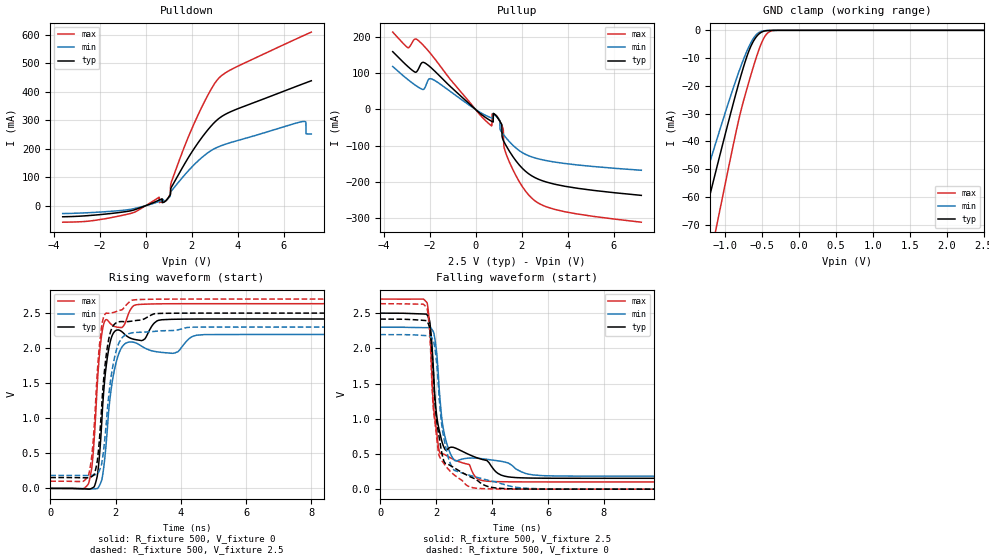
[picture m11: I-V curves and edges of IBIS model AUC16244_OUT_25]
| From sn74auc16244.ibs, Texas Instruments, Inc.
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[Model]   AUC16244_OUT_25
Model_type  3-state
Enable   Active-Low
Vref =   0
Rref =   500
Cref =   30p
Vmeas =   1.25
| variable   typ   min   max
C_comp   5.24pF   4.67pF   5.46pF
| C_pullup   7.75pF   4.60pF   11.92pF
| C_pulldown   6.72pF   4.63pF   15.60pF
| C_tri-state   5.24pF   4.67pF   5.46pF
[Temperature Range]   40   100   -40
| Ambient temperature   25   85   -40
[Voltage range]   2.5   2.3   2.7
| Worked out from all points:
|   slope of the pulldown table from 0 to 0.375 V, typ, clamps not added: 30.7 ohm
|   slope of the pullup table from 0 to 0.375 V, typ, clamps not added: 19 ohm
|   GND clamp passes 1 mA (typ) near -0.53 V on its own axis
|   rising waveform, R_fixture 500, V_fixture 0: 20-80 % time 261ps typ, 325ps min, 233ps max; typ from 0 V to 2.42 V
|   falling waveform, R_fixture 500, V_fixture 2.5: 20-80 % time 397ps typ, 379ps min, 287ps max; typ from 2.5 V to 0.154 V
|   rising waveform, R_fixture 500, V_fixture 2.5: 20-80 % time 262ps typ, 325ps min, 233ps max; typ from 0.154 V to 2.5 V
|   falling waveform, R_fixture 500, V_fixture 0: 20-80 % time 364ps typ, 416ps min, 295ps max; typ from 2.42 V to 0 V
[GND Clamp]
| AUC16244_OUT_25
|   Voltage   I(typ)   I(min)   I(max)
-3.6V     -322.9mA   -271.3mA   -392.8mA
-1.455V   -86.41mA   -69.74mA   -115.3mA
-1.345V   -74.46mA   -59.86mA   -100.9mA
-1.295V   -69.05mA   -55.41mA   -94.31mA
-1.105V   -48.71mA   -38.79mA   -69.37mA
-850mV    -22.51mA   -17.75mA   -36.48mA
-725mV    -11.06mA   -8.768mA   -23.02mA
-625mV    -4.339mA   -3.267mA   -13.84mA
-520mV    -878.8uA   -491uA     -5.429mA
-430mV    -104.5uA   -60.64uA   -1.111mA
-325mV    -4.915uA   -5.536uA   -43.94uA
2.5V      1.045nA    211.8nA    1.502nA
[Pulldown]
| AUC16244_OUT_25
|   Voltage   I(typ)   I(min)   I(max)
-3.6V     -38.75mA   -27.46mA   -57.79mA
-1.14V    -23.79mA   -17.18mA   -36mA
590mV     19.92mA    14.98mA    30.03mA
600mV     20.28mA    15.25mA    11.17mA
910mV     20.16mA    20.33mA    19.24mA
1.07V     37.88mA    45.66mA    41.07mA
1.915V    176.4mA    127.8mA    252.5mA
3.135V    303.2mA    205.9mA    444mA
6.825V    427.7mA    295.8mA    596.2mA
6.965V    431.9mA    293mA      601.3mA
6.97V     432.1mA    252.7mA    601.5mA
7.2V      439mA      251.9mA    609.9mA
[Pullup]
| AUC16244_OUT_25
|   Voltage   I(typ)   I(min)   I(max)
-3.6V     160mA      119mA      214.2mA
-2.935V   118.6mA    82.49mA    170.9mA
-2.405V   122.6mA    58.64mA    186.2mA
-1.88V    112.5mA    83.79mA    148.8mA
670mV     -31.69mA   -22.93mA   -44.2mA
720mV     -33.47mA   -24.18mA   -12.23mA
935mV     -20.74mA   -21.43mA   -18.64mA
1.19V     -83.17mA   -67.47mA   -51.41mA
1.235V    -89.46mA   -71.21mA   -103.5mA
1.49V     -117.6mA   -90.51mA   -148.5mA
2.565V    -188.1mA   -133.7mA   -252.1mA
7.2V      -237.7mA   -168.2mA   -311.9mA
[Ramp]
| AUC16244_OUT_25
| variable   typ   min   max
dV/dt_r   1.46/2.69E-10   1.32/3.31E-10   1.58/2.41E-10
dV/dt_f   1.41/4.04E-10   1.27/3.80E-10   1.56/2.90E-10
R_load = 500
[Rising Waveform]
| AUC16244_OUT_25
R_fixture =   500
C_fixture =   0
L_fixture =   0
V_fixture =   0
V_fixture_min = 0
V_fixture_max = 0
|   Time   V(typ)   V(min)   V(max)
0s        12.33nV    36.82nV    2.005nV
1.175ns   -10.36mV   -6.173mV   70.51mV
1.31ns    11.17mV    -6.967mV   475.7mV
1.485ns   353.8mV    22.7mV     1.785V
1.675ns   1.585V     453mV      2.391V
1.865ns   2.138V     1.411V     2.34V
2.17ns    2.243V     1.995V     2.294V
2.64ns    2.119V     2.071V     2.619V
3.73ns    2.411V     1.927V     2.633V
34.99ns   2.416V     2.195V     2.634V
[Falling Waveform]
| AUC16244_OUT_25
R_fixture =   500
C_fixture =   0
L_fixture =   0
V_fixture =   2.5
V_fixture_min = 2.3
V_fixture_max = 2.7
|   Time   V(typ)   V(min)   V(max)
0s        2.5V       2.3V       2.7V
1.675ns   2.475V     2.294V     2.646V
1.8ns     2.273V     2.291V     2.082V
1.93ns    1.474V     2.187V     1.074V
2.115ns   826.5mV    1.382V     531.7mV
2.29ns    583.4mV    786.6mV    493.4mV
2.59ns    595.4mV    442.5mV    428.8mV
3.65ns    421.9mV    432.1mV    121.9mV
5.205ns   159.2mV    222.4mV    103.2mV
34.99ns   154.5mV    184.4mV    102.7mV
[Rising Waveform]
| AUC16244_OUT_25
R_fixture =   500
C_fixture =   0
L_fixture =   0
V_fixture =   2.5
V_fixture_min = 2.3
V_fixture_max = 2.7
|   Time   V(typ)   V(min)   V(max)
0s        154.5mV    184.4mV    102.6mV
1.175ns   151.5mV    183.1mV    189.6mV
1.305ns   180.3mV    188mV      624.3mV
1.465ns   487mV      217.7mV    1.813V
1.615ns   1.439V     474.5mV    2.409V
1.825ns   2.197V     1.457V     2.499V
2.095ns   2.375V     2.066V     2.535V
2.525ns   2.387V     2.22V      2.686V
3.875ns   2.498V     2.258V     2.7V
34.99ns   2.5V       2.3V       2.7V
[Falling Waveform]
| AUC16244_OUT_25
R_fixture =   500
C_fixture =   0
L_fixture =   0
V_fixture =   0
V_fixture_min = 0
V_fixture_max = 0
|   Time   V(typ)   V(min)   V(max)
0s        2.416V     2.195V     2.634V
1.675ns   2.382V     2.179V     2.568V
1.795ns   2.205V     2.172V     2.019V
1.92ns    1.484V     2.077V     1.062V
2.1ns     752.2mV    1.333V     482.2mV
2.24ns    446.1mV    798.6mV    383.9mV
2.52ns    332.6mV    350.4mV    247mV
3.315ns   158.9mV    183.4mV    20.07mV
5.96ns    541.9uV    3.344mV    108uV
34.99ns   29.54uV    1.853uV    13.72uV
